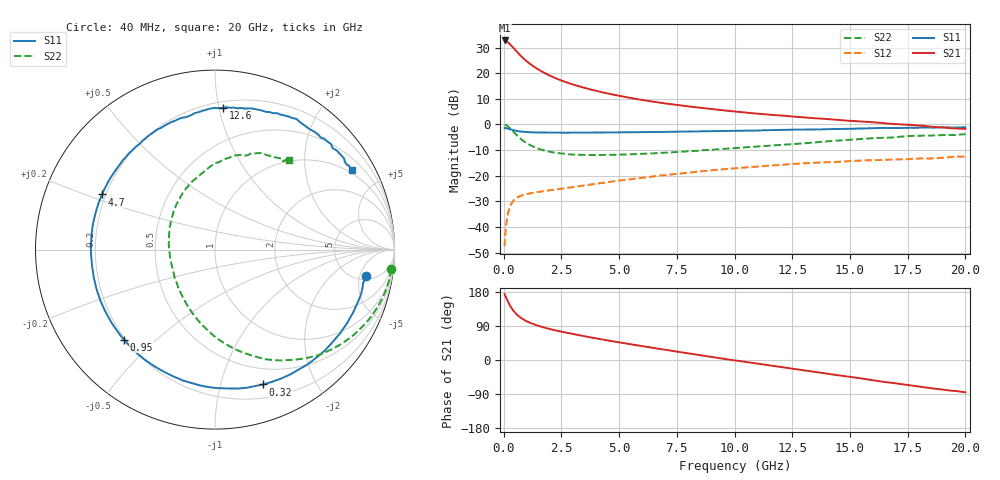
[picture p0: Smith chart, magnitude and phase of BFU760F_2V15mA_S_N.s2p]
! Filename:  P:\Prog\Test\Noise\ATS_data\Testdata_Net\BFU760\BFU760F_2W_C1_2V15mA_D.s2p
! Date/Time: Mon 06/Feb/2012 15:05:30
! BFU760_2W_C1_2V15mA
! bias mode 1: Vout= 2.0001 V, Iout=15.0350 mA, Vin= 0.7818 V, Iin= 0.0455 mA
! Date/time Fri Mar 18 13:53:57 2011
! Device data file deembeded for feedlines and parallel
! Original file: \BFU760\BFU760_2W_C1_2V15mA_R.s2p
! Feed-files: PR003V01_101208_Feed1.s2p, PR003V01_101208_Feed2.s2p
! Parallel-file: PR003V01_101208_Par.s2p
# MHz S MA R 50
!  Freq-MHz  S11-mag  S11-arg  S21-mag  S21-arg  S12-mag  S12-arg  S22-mag  S22-arg
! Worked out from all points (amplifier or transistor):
!   167 points, 40 MHz to 20 GHz, reference 50 ohm
!   highest |S21| = 32.8 dB at 40 MHz (marker M1)
!   |S21| within 3 dB of that: start of sweep to 430.5 MHz
!   unconditionally stable (mu >= 1): 4.72 GHz to 13.66 GHz
!   at 550 MHz: K = 0.19, MSG = 28.7 dB, |S12| = -28.7 dB
!   at 4.2 GHz: K = 0.96, MSG = 17.8 dB, |S12| = -22.9 dB
!   at 20 GHz: K = 0.87, MSG = 5.4 dB, |S12| = -12.5 dB
!   lowest NFmin = 0.47 dB at 400 MHz
!   S11 on the Smith chart (normalised r, x): 40 MHz: 5.84, -6.27; 320 MHz: 0.33, -1.37; 950 MHz: 0.19, -0.40; 4.7 GHz: 0.19, +0.22; 12.6 GHz: 0.24, +1.03; 20 GHz: 0.87, +3.52
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40  0.8536 -9.8  43.51 174.2  0.004234 83.2  0.9885 -6.4
50  0.8461 -12.9  43.43 172.1  0.00539 87.2  0.9855 -8.2
120  0.8423 -29.0  41.95 162.6  0.01236 75.5  0.9595 -19.8
180  0.8311 -42.5  40.06 154.8  0.01784 69.0  0.9198 -29.0
240  0.8148 -55.3  38.03 147.5  0.02254 63.3  0.873 -37.6
320  0.7977 -70.4  34.89 139.2  0.02767 56.5  0.804 -48.0
400  0.7786 -83.8  31.96 131.9  0.03161 51.1  0.7356 -56.8
480  0.7636 -94.8  29.01 125.9  0.03468 46.6  0.6761 -64.8
600  0.7428 -108.8  25.34 118.3  0.03794 41.7  0.5953 -74.7
750  0.7277 -122.2  21.57 111.0  0.04082 37.4  0.5189 -85.0
950  0.7141 -135.3  17.82 103.7  0.04346 34.0  0.4449 -96.2
1300  0.7013 -151.1  13.51 94.4  0.04676 31.0  0.3658 -111.7
1850  0.693 -166.7  9.683 83.9  0.05095 29.9  0.3038 -129.9
2500  0.6917 -178.9  7.198 74.7  0.05599 30.4  0.2727 -146.1
3400  0.694 168.6  5.328 63.9  0.06411 30.7  0.256 -162.4
4700  0.7007 154.0  3.856 49.6  0.07734 29.9  0.2559 178.6
6800  0.7155 134.1  2.652 28.9  0.1009 24.5  0.2787 155.0
10200  0.7553 105.7  1.758 -2.8  0.1419 9.2  0.3518 123.2
12600  0.7907 86.8  1.417 -23.8  0.1701 -4.3  0.4164 103.3
13400  0.7969 81.1  1.331 -30.6  0.1789 -9.9  0.4435 97.1
16800  0.853 54.9  1.029 -60.2  0.2061 -31.1  0.558 70.7
20000  0.8833 30.1  0.822 -85.4  0.2361 -52.8  0.6459 50.5
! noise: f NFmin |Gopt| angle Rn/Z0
400  0.4712  0.06696  76.67  0.0525
650  0.4741  0.0944  99.61  0.0511
1050  0.4809  0.1432  117.6  0.0489
1450  0.4904  0.1888  128.3  0.0468
1850  0.5025  0.2299  136.8  0.0448
2300  0.5193  0.2719  145.4  0.0426
2900  0.5471  0.3233  156.1  0.04
3700  0.5933  0.3897  170  0.0369
4500  0.6503  0.4599  183.1  0.0346
6000  0.7859  0.6094  205.1  0.0324
